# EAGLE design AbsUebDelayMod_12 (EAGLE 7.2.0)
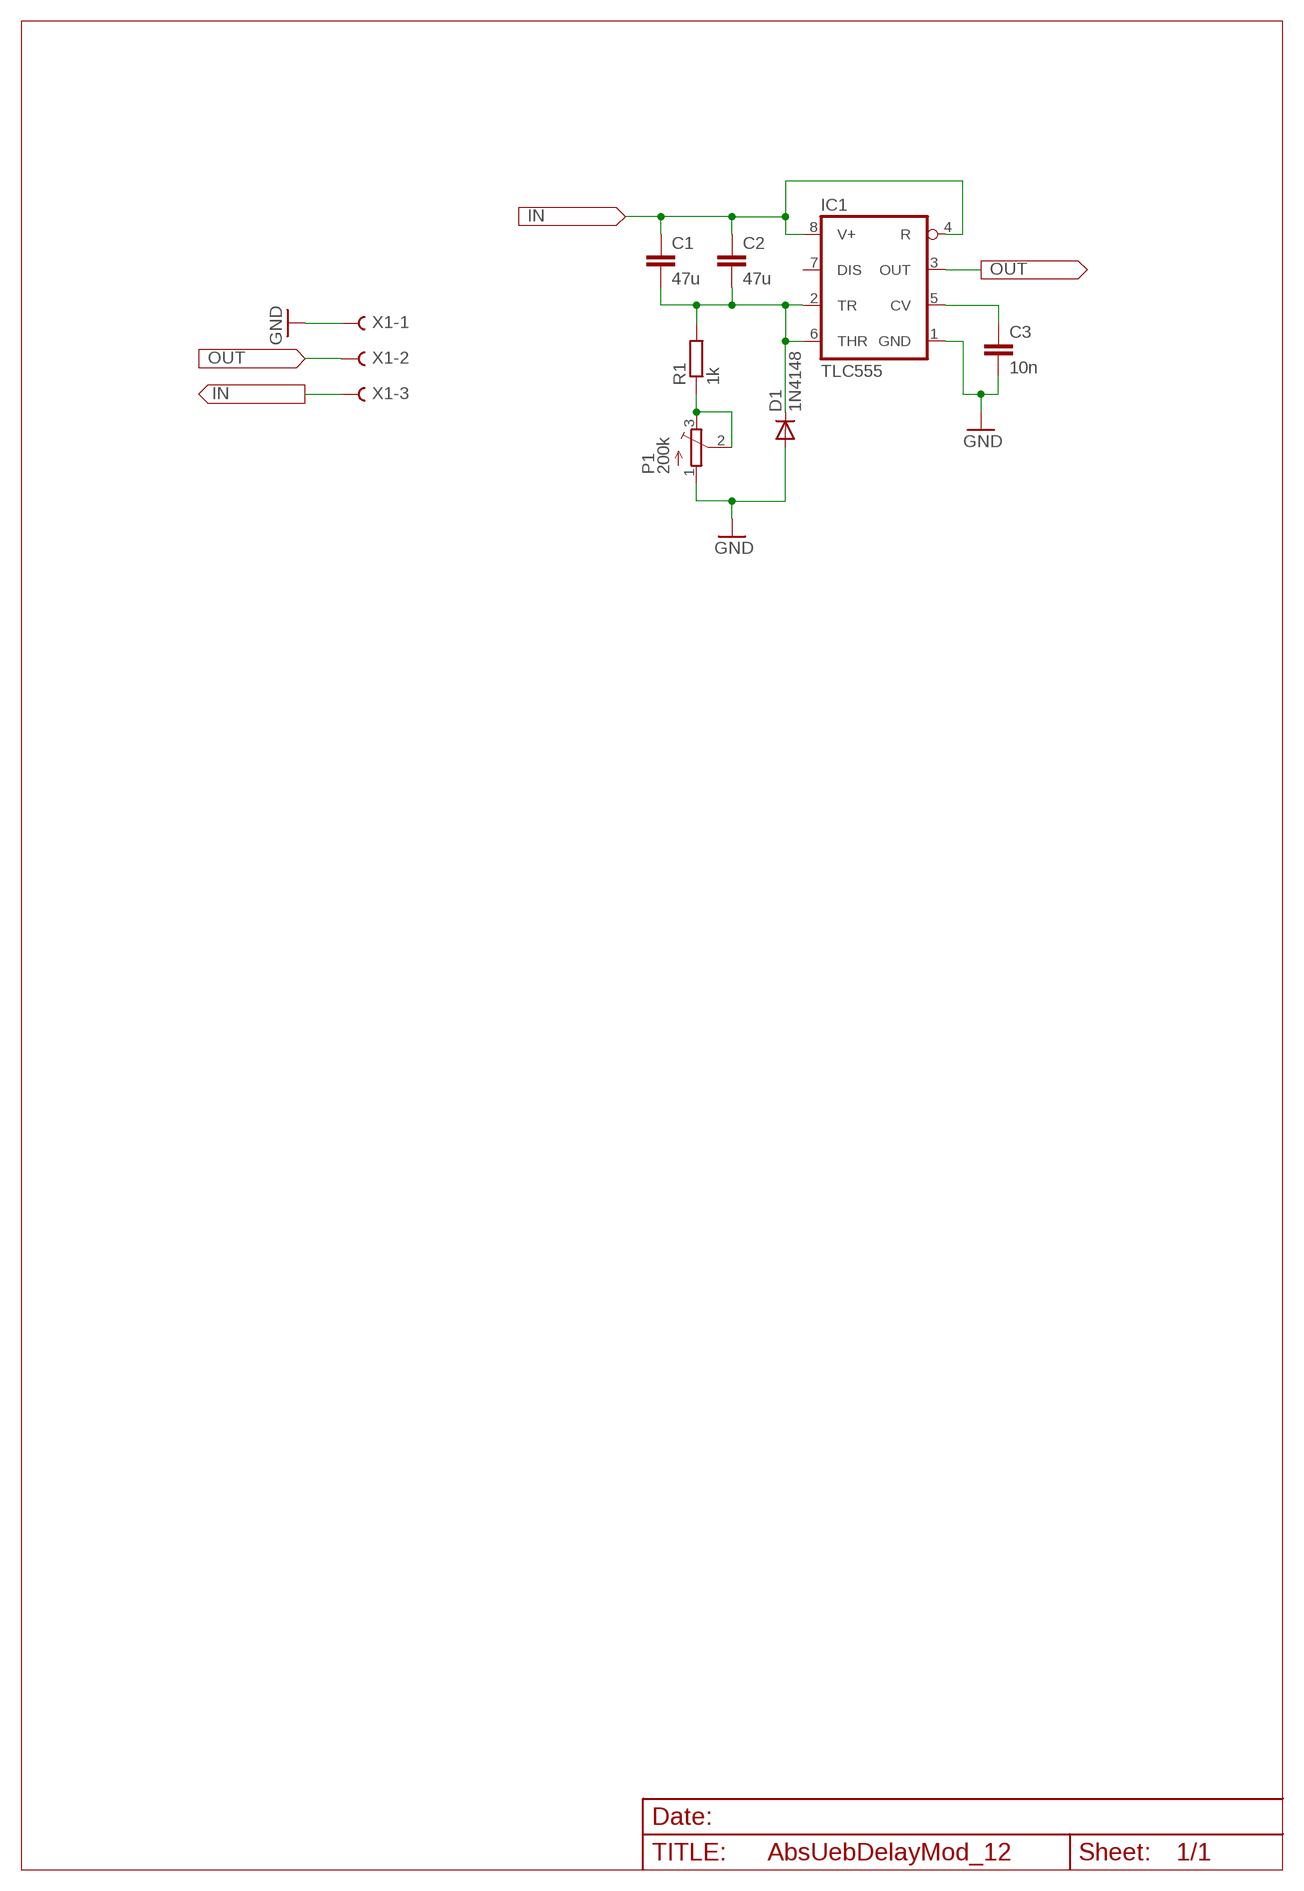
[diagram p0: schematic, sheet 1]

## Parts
C1  47u  C-SMD-1210  [C1210]
C2  47u  C-SMD-1210  [C1210]
C3  10n  C-SMD-1206  [C1206]
D1  1N4148  [SOD80-LL34]
IC1  TLC555  [SOIC08]
P1  200k  TRIM_23B-200KM23  [MODEL23]
R1  1k  R-SMD-1206  [R1206]
X1  PINFE-1X03  [PINFE-1X03_LOCK]

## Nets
GND: C3.2 D1.2(A) IC1.1(GND) P1.1(A) X1.1
IN: C1.1 C2.1 IC1.4(R) IC1.8(V+) X1.3
N$1: C1.2 C2.2 D1.1(C) IC1.2(TR) IC1.6(THR) R1.2
N$3: P1.2(S) P1.3(E) R1.1
N$11: C3.1 IC1.5(CV)
OUT: IC1.3(OUT) X1.2
Unconnected: IC1.7(DIS)

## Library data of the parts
C1-C3 = AbsUebParts_11:C-SMD: SMD Keramik Vielschichtkondensatoren
D1 = AbsUebParts_11:1N4148: 1N4148 Diode; MF: Vishay; MPN: LL4148; OC_REICHELT: 1N 4148 SMD
IC1 = AbsUebParts_11:*555: TIMER NE555 compatible general purpose timer IC; MF: TI; MPN: TLC555CD; OC_REICHELT: TLC 555 CD SMD
P1 = AbsUebParts_11:TRIM_23B-200K: POTENTIOMETER; MF: BI Technologies; MPN: 23BR200KLFTR; OC_REICHELT: 23B-200K
R1 = AbsUebParts_11:R-SMD: SMD Resistor
X1 = AbsUebParts_11:PINFE-1X03: FEMALE CONNECTOR 1X3 RM 2.54 mm; MF: MPE-GARRY; MPN: 094-1-003-0-NFX-YS0; OC_REICHELT: MPE 094-1-003

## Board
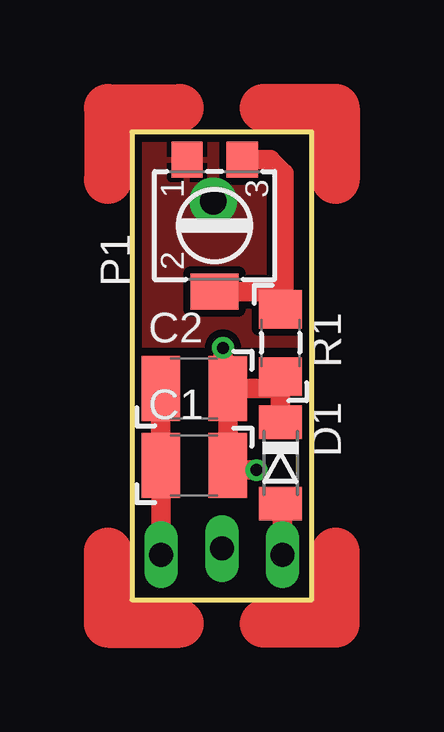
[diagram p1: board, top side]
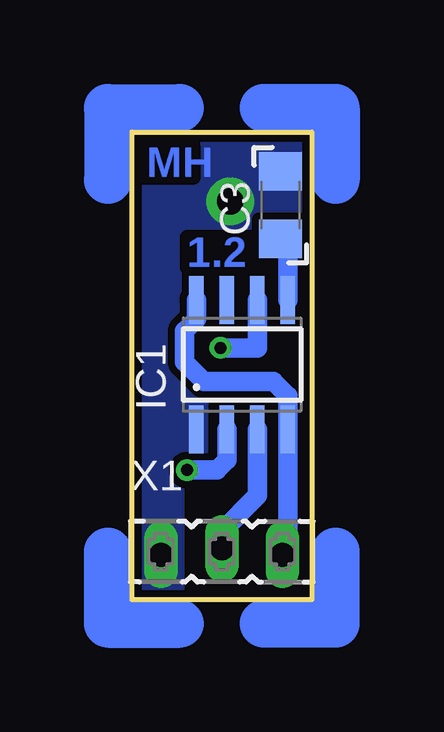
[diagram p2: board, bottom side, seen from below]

Size 7.5 x 19.5 mm. Coordinates in mm from the lower left corner, seen from the top.
Outline: 0,0 7.5,0 7.5,19.5 0,19.5 0,0
Copper layers (1*16): Top 0.035mm / dielectric 1.5mm / Bottom 0.035mm
Design rules "PCB-POOL Standard *": minimum track width 0.15mm, minimum drill 0.3mm, track to track 0.15mm, track to pad 0.15mm, pad to pad 0.15mm, via to via 0.15mm, smd to smd 0.15mm, copper to edge 0.3mm, drill to drill 0.2mm, minimum pad ring 0.2mm, minimum via ring 0.15mm, stop-mask expansion 0.075mm, vias tented up to drill 20mil, thermal gap 0.2mm

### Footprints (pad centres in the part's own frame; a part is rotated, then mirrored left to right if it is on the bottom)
C1210 = smd 1.6 x 2.7: 1 -1.4,0; 2 1.4,0
C1206 = smd 1.6 x 1.8: 1 -1.4,0; 2 1.4,0
SOD80-LL34 = smd 1.4 x 1.8: 1 -1.7,0; 2 1.7,0
SOIC08 = smd 0.6 x 2: 1 -1.905,-2.7; 2 -0.635,-2.7; 3 0.635,-2.7; 4 1.905,-2.7; 5 1.905,2.7; 6 0.635,2.7; 7 -0.635,2.7; 8 -1.905,2.7
MODEL23 = smd 1.5 x 1.3: 1 2.75,1.15; 3 2.75,-1.15 | smd 1.5 x 2: 2 -2.75,0
R1206 = smd 1.6 x 1.8: 1 -1.4,0; 2 1.4,0
PINFE-1X03_LOCK = drill 1 long: 1 -2.54,-0.127; 2 0,0.127; 3 2.54,-0.127

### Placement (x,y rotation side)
C1  2.6,5.6 0 top
C2  2.6,8.8 0 top
C3  1.3,16.45 90 bottom
D1  6.2,5.7 270 top
DRILEGEND  [DRILEGEND]  not placed on the board
IC1  2.9,9.8 0 bottom
P1  3.45,15.6 90 top
R1  6.2,10.7 270 top
X1  3.75,2 0 bottom

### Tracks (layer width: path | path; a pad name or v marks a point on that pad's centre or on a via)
GND  (via drill 1.1)
  Top 0.813: D1.2 6.29,4.02 X1.1
  other vias: 3.4,16.6
  pour Top (isolate 0.305): 0,10.6 0,19.5 7.5,19.5 7.5,10.6
  pour Bottom (isolate 0.305, no thermals): 5.4,0 5.4,5 4.4,5 4.4,10 0,10 0,19.5 7.5,19.5 7.5,0
IN
  Top 0.813: X1.3 C1.1 C2.1
  Bottom 0.813: IC1.8 4.8,11.7 5.3,11.2 5.3,9.9 4.5,9.1 1.6,9.1 0.99,8.49 IC1.4 0.99,2.09 X1.3
N$1  (via drill 0.5)
  Top 0.813: C2.2 C1.2 4,5.4 v5.2,5.4 | C2.2 3.6,9.2 3.8,9.4 v3.8,10.5 | C2.2 6.2,8.8 R1.2 D1.1
  Bottom 0.813: v3.8,10.5 2.27,10.5 IC1.6 | v5.2,5.4 3.95,5.4 3.54,5.82 IC1.2
N$2
  Top 2: 2,-1 -1,-1 -1,2
N$3
  Top 0.813: P1.3 5.78,18.35 6.35,17.78 6.35,13 6.35,12.85 | P1.2 6.35,12.85 | R1.1 6.35,12.1 6.35,12.85
N$4
  Bottom 2: 2,-1 -1,-1 -1,2
N$5
  Top 2: -1,17.5 -1,20.5 2,20.5
N$6
  Bottom 2: -1,17.5 -1,20.5 2,20.5
N$7
  Top 2: 5.5,20.5 8.5,20.5 8.5,17.5
N$8
  Bottom 2: 5.5,20.5 8.5,20.5 8.5,17.5
N$9
  Top 2: 8.5,2 8.5,-1 5.5,-1
N$10
  Bottom 2: 8.5,2 8.5,-1 5.5,-1
N$11
  Bottom 0.813: IC1.5 0.99,15.2 C3.1
OUT
  Bottom 0.813: IC1.3 2.27,4.33 3.75,2.85 X1.2

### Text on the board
Bottom: MH | 1.2
DrillLegend: LAYER-STACK
DrillLegend_01-16: 01-16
